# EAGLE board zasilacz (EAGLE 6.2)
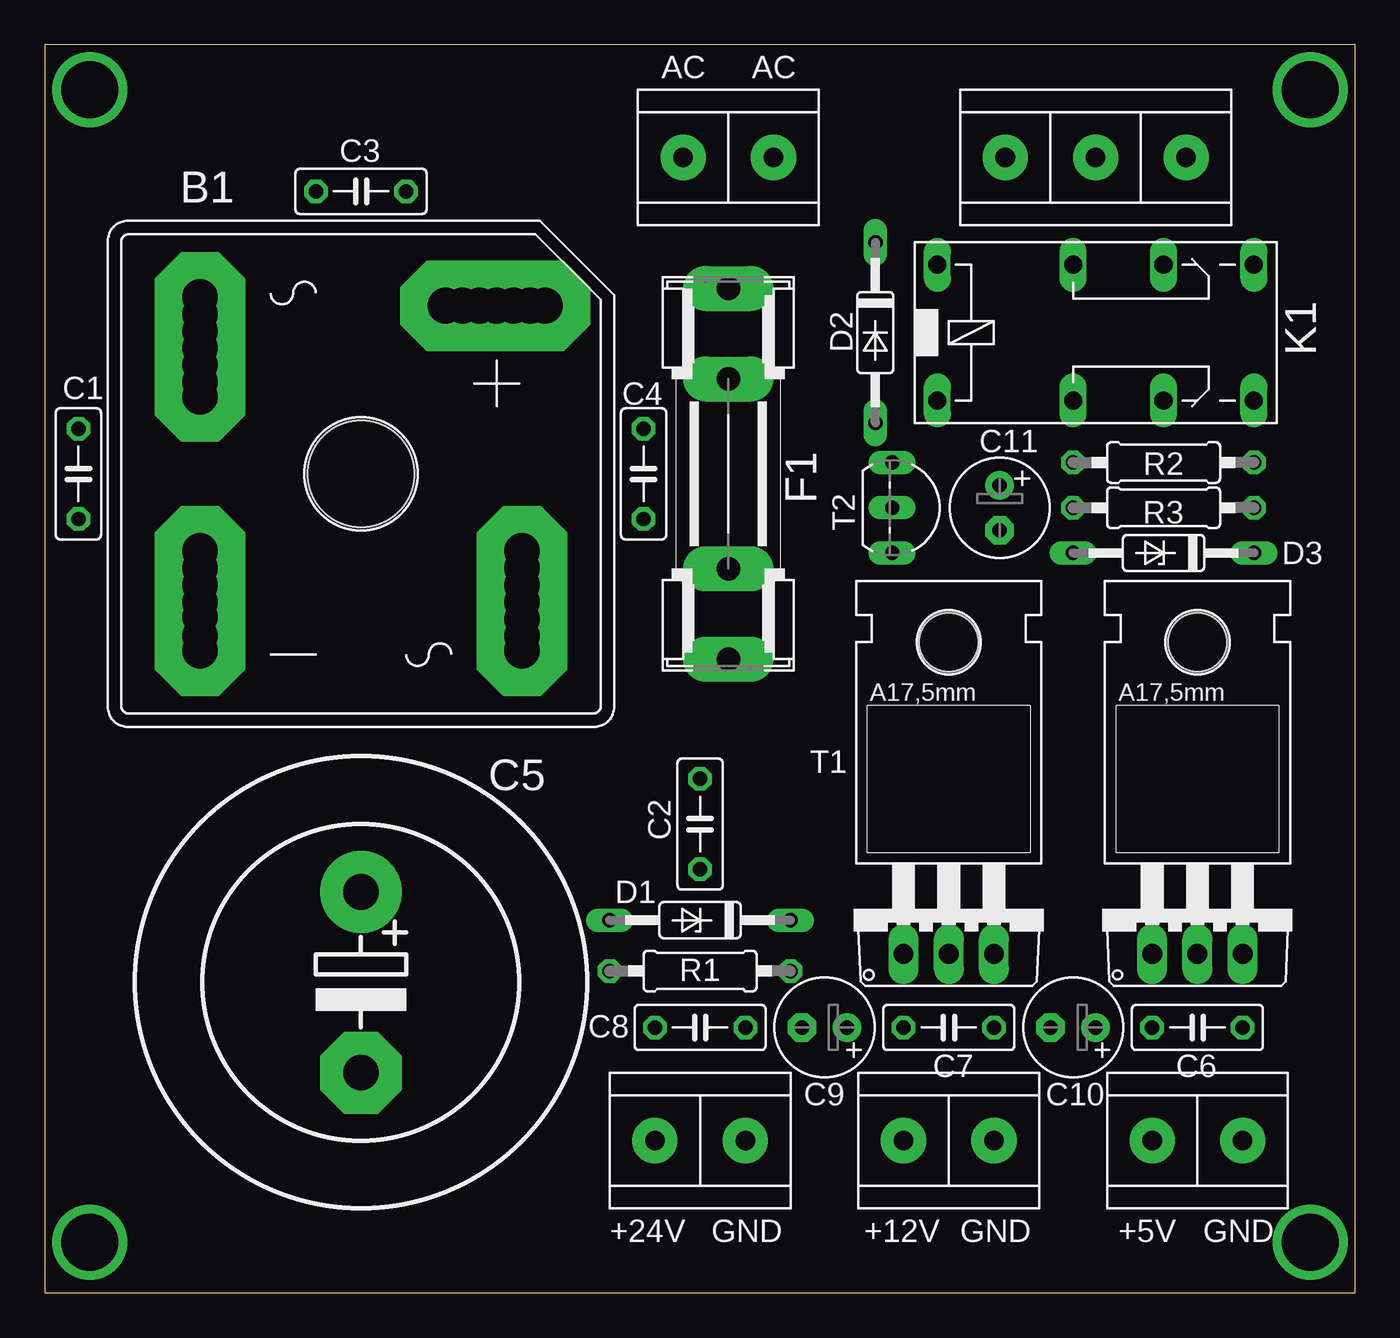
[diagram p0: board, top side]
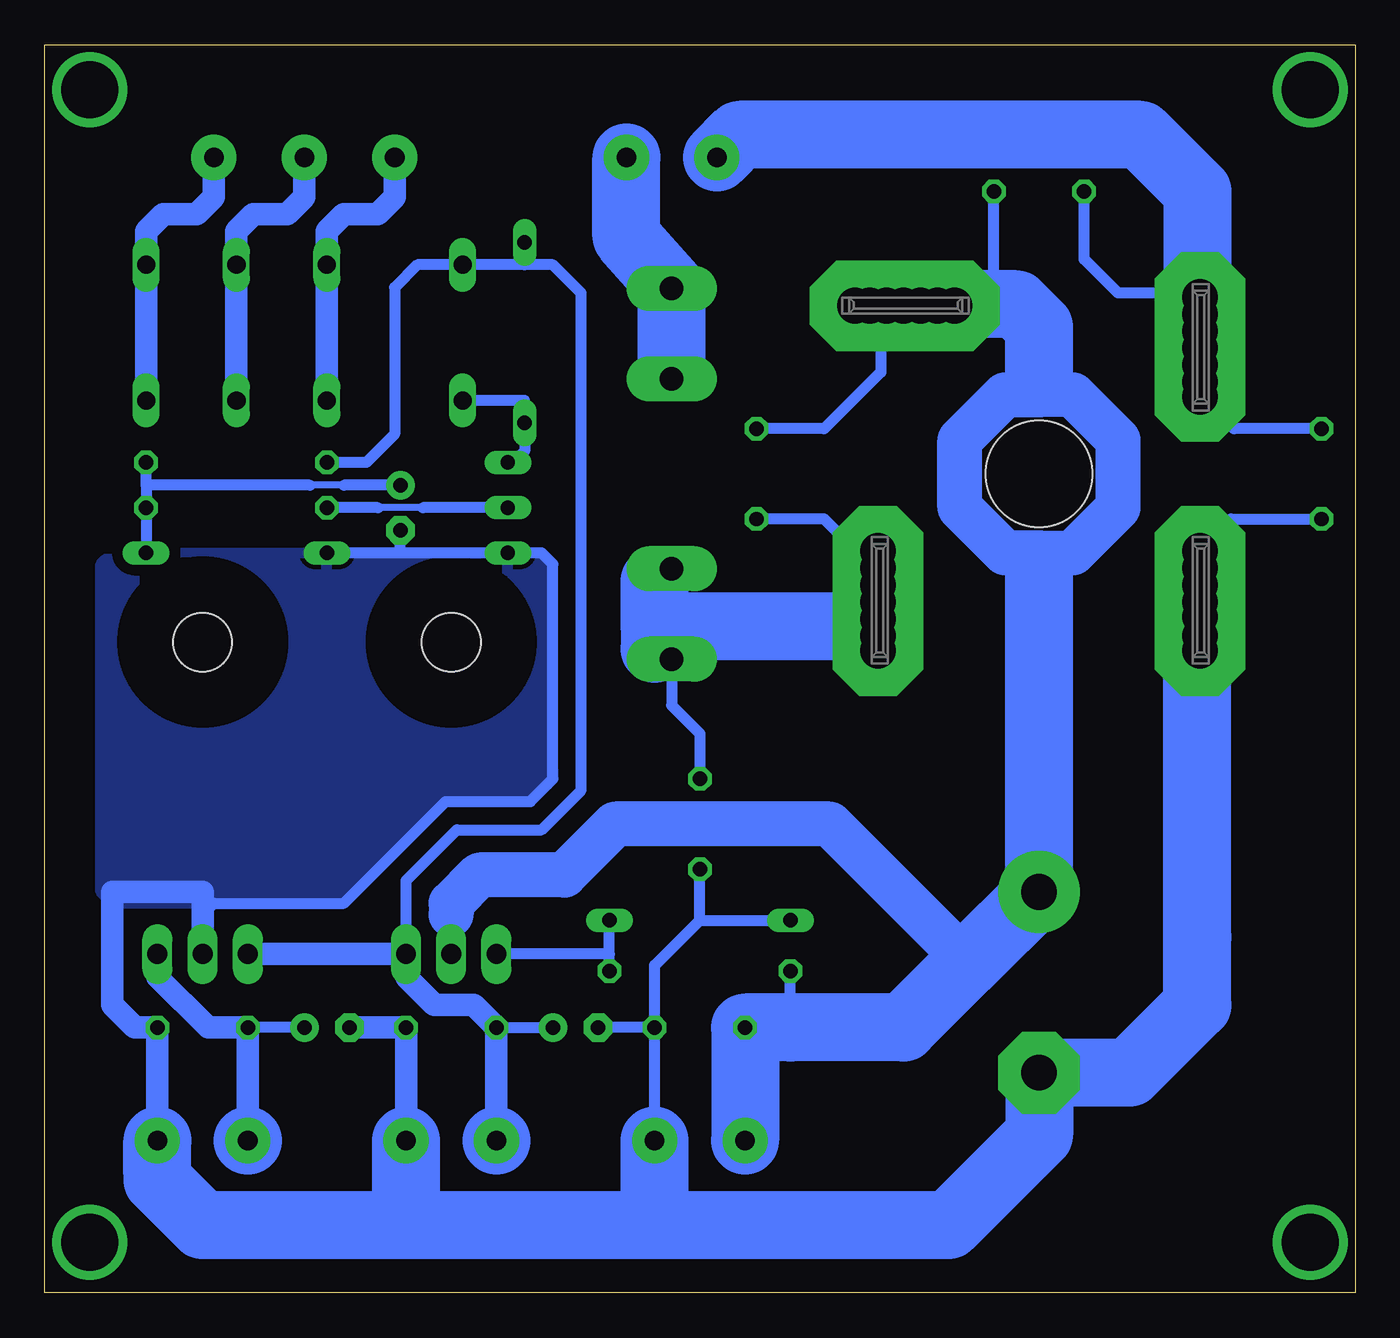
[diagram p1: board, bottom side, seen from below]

Size 73.65 x 70.16 mm. Coordinates in mm from the lower left corner, seen from the top.
Outline: 0,70.16 0,0 73.65,0 73.65,70.16 0,70.16
Copper layers (1*16): Top 0.035mm / dielectric 1.5mm / Bottom 0.035mm
Design rules: minimum track width 10mil, minimum drill 24mil, track to track 8mil, track to pad 8mil, pad to pad 8mil, via to via 8mil, smd to smd 8mil, copper to edge 40mil, drill to drill 8mil, minimum pad ring 10mil, minimum via ring 8mil, stop-mask expansion 4mil, vias tented up to drill 0mil, thermal gap 10mil

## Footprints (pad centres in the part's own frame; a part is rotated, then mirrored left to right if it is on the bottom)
B25A- = drill 2.007 pad 5.08 octagon: + 10.338,9.449; +1 4.75,9.449; +2 6.655,9.449; +3 8.56,9.449; +4 5.702,9.449; +5 7.607,9.449; +6 9.512,9.449; - -9.042,-4.343; -1 -9.042,-9.931; -2 -9.042,-8.026; -3 -9.042,-6.248; -4 -9.042,-5.296; -5 -9.042,-7.201; -6 -9.042,-9.106; AC1 -9.042,4.343; AC1- -9.042,9.931; AC1-1 -9.042,8.026; AC1-2 -9.042,6.121; AC1-3 -9.042,8.979; AC1-4 -9.042,7.074; AC1-5 -9.042,5.169; AC2 9.042,-4.343; AC2- 9.042,-9.931; AC3 9.042,-6.248; AC4 9.042,-8.153; AC5 9.042,-7.201; AC6 9.042,-5.296; AC7 9.042,-9.106 | hole 6: 0,0
C050-025X075 = drill 0.813 octagon: 1 -2.54,0; 2 2.54,0
EB25D = drill 2.007 pad 4.597: + -5.08,0 | drill 2.007 pad 4.597 octagon: - 5.08,0
E2,5-6 = drill 0.813 pad 1.6: + -1.27,0 | drill 0.813 pad 1.6 octagon: - 1.27,0
DO35Z10 = drill 0.813 long: A 5.08,0; C -5.08,0
DO35-10 = drill 0.813 long: A 5.08,0; C -5.08,0
SHK20L = drill 1.321 pad 2.54 long: 1A -10.414,0; 1B -5.334,0; 2A 10.414,0; 2B 5.334,0
351 = drill 1.016 long: 1 -3.81,-3.81; 16 -3.81,3.81; O1 8.89,-3.81; O2 8.89,3.81; P1 3.81,-3.81; P2 3.81,3.81; S1 13.97,-3.81; S2 13.97,3.81
TO220 = drill 1.118 long: 1 -2.54,-6.35; 2 0,-6.35; 3 2.54,-6.35 | hole 3.302: 0,11.176
0207/10 = drill 0.813 octagon: 1 -5.08,0; 2 5.08,0
TO220AV = drill 1.016 long: B -2.54,-2.54; C 0,-2.54; E 2.54,-2.54
TO92-EBC = drill 0.813 long: B 0,-1.27; C -2.54,-1.27; E 2.54,-1.27
TO220V = drill 1.016 long: 1 -2.54,-2.54; 2 0,-2.54; 3 2.54,-2.54
ARK2 = drill 1.1 pad 2.54: P$1 -2.54,0; P$2 2.54,0
AREK3 = drill 1.1 pad 2.54: P$1 0,0; P$2 -5.08,0; P$3 5.08,0

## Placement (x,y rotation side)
B1  [B25A-]  17.78,46.02 0 top
C1  [C050-025X075]  1.9,46.02 270 top
C2  [C050-025X075]  36.83,26.34 270 top
C3  [C050-025X075]  17.78,61.9 0 top
C4  [C050-025X075]  33.65,46.02 270 top
C5  [EB25D]  17.78,17.45 270 top
C6  [C050-025X075]  64.77,14.91 0 top
C7  [C050-025X075]  50.8,14.91 0 top
C8  [C050-025X075]  36.83,14.91 0 top
C9  [E2,5-6]  43.81,14.91 180 top
C10  [E2,5-6]  57.78,14.91 180 top
C11  [E2,5-6]  53.66,44.12 270 top
D1  [DO35Z10]  36.83,20.94 180 top
D2  1N4446  [DO35-10]  46.67,53.96 270 top
D3  [DO35Z10]  62.87,41.58 180 top
F1  [SHK20L]  38.42,46.02 270 top
K1  351  [351]  53.97,53.96 0 top
Q1  2N6101  [TO220]  50.8,25.39 0 top
Q2  2N6101  [TO220]  64.77,25.39 0 top
R1  [0207/10]  36.83,18.08 180 top
R2  [0207/10]  62.87,46.66 0 top
R3  [0207/10]  62.87,44.12 180 top
T1  BD649  [TO220AV]  50.8,21.58 0 top
T2  BC447  [TO92-EBC]  48.89,44.12 270 top
U1  7805  [TO220V]  64.77,21.58 0 top
U$1  ARK2  [ARK2]  38.42,63.8 0 top
U$2  ARK2  [ARK2]  50.8,8.56 180 top
U$3  ARK2  [ARK2]  64.77,8.56 180 top
U$4  ARK2  [ARK2]  36.83,8.56 180 top
U$5  AREK3  [AREK3]  59.05,63.8 0 top

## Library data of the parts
B1 = rectifier
C1-C11 R1-R3 = rcl
D1-D3 = diode
F1 = fuse
K1 = relay
Q1 Q2 T2 = transistor-npn
T1 = transistor-power
U1 = linear
U$1-U$4 = arek2
U$5 = arek3

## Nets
GND: B1.-1 C1.2 C2.2 C5.- C6.2 C7.2 C8.2 C9.- C10.- C11.- D1.A D3.A T2.E U1.2 U$2.P$1 U$3.P$1 U$4.P$1
N$1: B1.AC1- C1.1 C3.1 U$1.P$1
N$2: B1.AC2- C2.1 C4.2 F1.2A
N$3: F1.1A U$1.P$2
N$5: K1.O1 K1.O2 U$5.P$1
N$6: D1.C R1.1 T1.B
N$7: C6.1 C10.+ U1.3 U$3.P$2
N$8: B1.+1 C3.2 C4.1 C5.+ C8.1 R1.2 T1.C U$4.P$2
N$14: D2.A K1.1 T2.C
N$15: R3.2 T2.B
N$16: C11.+ D3.C R2.2 R3.1
N$17: C7.1 C9.+ D2.C K1.16 R2.1 T1.E U1.1 U$2.P$2
N$18: K1.S1 K1.S2 U$5.P$3
N$19: K1.P1 K1.P2 U$5.P$2

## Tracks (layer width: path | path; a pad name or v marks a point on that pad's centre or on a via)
GND
  Bottom 0.61: C1.2 6.99,43.48 8.89,41.58 8.89,35.23 | 8.74,32.21 8.74,20.78 8.89,19.99 | 53.97,3.8 53.34,4.12 53.34,5.07 54.61,3.8 | C8.2 C9.- | C8.2 39.37,18.4 36.83,20.94 | U$4.P$1 C8.2 | 36.83,20.94 C2.2 | 36.83,20.94 D1.A | 53.66,41.58 T2.E 45.72,41.58 45.08,40.95 45.08,28.88 46.35,27.61 51.12,27.61 56.83,21.89 64.14,21.89 64.77,21.26 | 53.66,41.58 D3.A | 53.66,41.58 C11.-
  Bottom 1.27: U$2.P$1 C7.2 C10.- | U1.2 64.77,21.26 64.77,22.53 69.85,22.53 69.85,16.18 68.58,14.91 C6.2 U$3.P$1 | 67.31,6.34 67.31,6.66 66.99,6.34 67.31,6.34 | 67.31,6.34 67.31,6.02
  Bottom 2.54: 8.74,32.21 B1.-1 | 53.97,3.8 53.97,7.29 U$2.P$1
  Bottom 3.81: 53.34,3.8 53.34,5.07 U$2.P$1 | 39.37,3.8 U$4.P$1 | 8.89,37.13 8.89,35.23 8.89,19.99 8.89,16.18 12.7,12.37 C5.- 17.78,8.88 22.86,3.8 39.37,3.8 | 39.37,3.8 53.34,3.8 | 53.34,3.8 53.97,3.8 54.61,3.8 64.77,3.8 67.31,6.34 | 67.31,6.66 U$3.P$1
  pour Bottom (isolate 0.61): 45.4,28.88 46.67,27.61 51.43,27.61 57.15,21.89 69.85,21.89 70.48,22.53 70.48,40.95 69.85,41.58 46.04,41.58 45.4,40.95 45.08,28.88 45.4,28.56
N$1
  Bottom 0.61: 8.74,50.47 B1.AC1- 8.97,56.18 13.34,56.18 15.24,58.09 C3.1 | 8.74,50.47 8.74,50.32 | C1.1 6.83,48.56 8.74,50.47
  Bottom 1.27: B1.AC1- 8.89,56.11
  Bottom 2.54: 8.89,61.9 8.89,56.11 8.89,51.1
  Bottom 3.81: 8.89,51.1 8.89,61.9 12.07,65.08 34.61,65.08 U$1.P$1
N$2
  Bottom 0.61: C4.2 29.84,43.48 26.67,40.31 26.67,36.25 B1.AC2- | 33.65,37.45 37.78,37.45 38.42,36.82 38.42,33.01 36.83,31.42 C2.1
  Bottom 1.27: 39.37,36.18 F1.2A | B1.AC2- 27.05,35.87 27.3,37.45
  Bottom 2.54: 39.37,39.99 39.37,39.67
  Bottom 3.81: 27.3,37.45 33.65,37.45 39.37,37.45 | 39.37,37.45 39.37,36.18 | 39.37,37.45 39.37,39.99
N$3
  Bottom 1.27: 38.42,56.5 F1.1A
  Bottom 3.81: U$1.P$2 40.96,59.36 38.42,56.5 38.42,52.38
N$4  (via drill 3.2)
  other vias: 2.54,67.62
N$5
  Bottom 1.27: K1.O1 K1.O2 62.87,59.68 61.91,60.63 60.01,60.63 59.05,61.58 U$5.P$1
N$6
  Bottom 0.61: 41.91,19.04 T1.B | R1.1 41.91,19.04 | 41.91,19.04 D1.C
N$7
  Bottom 0.61: C10.+ C6.1
  Bottom 1.27: U$3.P$2 C6.1 64.45,14.91 67.31,17.77 U1.3
N$8
  Bottom 0.61: C3.2 20.32,56.18 22.23,55.78 B1.+1 | 22.86,55.55 22.61,55.55 26.04,55.55 26.67,54.91 26.67,51.74 29.84,48.56 C4.1 | 50.8,21.26 T1.C | 31.75,14.91 R1.2
  Bottom 2.54: 17.78,40.95 17.78,41.58 | 17.78,41.58 19.68,41.58 22.23,44.12 22.23,47.93 19.68,50.47 17.78,50.47 | 17.78,41.58 15.88,41.58 13.34,44.12 13.34,47.93 15.88,50.47 17.78,50.47 | 17.78,50.47 17.78,51.1 | 19.05,55.55 22.45,55.55 B1.+1 22.61,55.55 | 50.8,21.26 50.8,21.89 49.21,23.48 44.45,23.48 41.59,26.34 29.53,26.34 21.75,18.56
  Bottom 3.81: 22.86,55.55 19.05,55.55 17.78,54.28 17.78,51.1 | 17.78,40.95 C5.+ 21.75,18.56 25.4,14.91 31.75,14.91 C8.1 U$4.P$2
N$9  (via drill 3.2)
  other vias: 71.12,67.62
N$10  (via drill 3.2)
  other vias: 2.54,2.85
N$11  (via drill 3.2)
  other vias: 71.12,2.85
N$14
  Bottom 0.61: K1.1 46.67,50.15 D2.A 46.67,47.3 47.31,46.66 T2.C
N$15
  Bottom 0.406: 52.39,44.12 54.93,44.12
  Bottom 0.61: T2.B 52.39,44.12 | 54.93,44.12 R3.2
N$16
  Bottom 0.406: 56.83,45.39 58.74,45.39
  Bottom 0.61: D3.C R3.1 67.95,45.39 | 67.95,45.39 R2.2 | C11.+ 56.83,45.39 | 58.74,45.39 67.95,45.39
N$17
  Bottom 0.61: C7.1 C9.+ | T1.E 53.34,23.16 50.48,26.02 45.72,26.02 43.5,28.24 43.5,54.6 43.5,56.18 45.08,57.77 46.67,57.77 | 46.67,57.77 K1.16 52.7,57.77 53.97,56.5 53.97,48.25 55.56,46.66 R2.1 | 46.67,57.77 D2.C
  Bottom 1.27: U1.1 T1.E 53.34,17.77 51.75,16.18 49.53,16.18 C7.1 U$2.P$2
N$18
  Bottom 1.27: K1.S1 K1.S2 67.95,59.68 66.99,60.63 65.09,60.63 64.14,61.58 U$5.P$3
N$19
  Bottom 1.27: K1.P1 K1.P2 57.78,59.68 56.83,60.63 54.93,60.63 53.97,61.58 U$5.P$2
(copper drawn outside any net)
  shapes: Bottom circle x2

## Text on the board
tPlace: AC | AC | +24V | GND | +12V | GND | +5V | GND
